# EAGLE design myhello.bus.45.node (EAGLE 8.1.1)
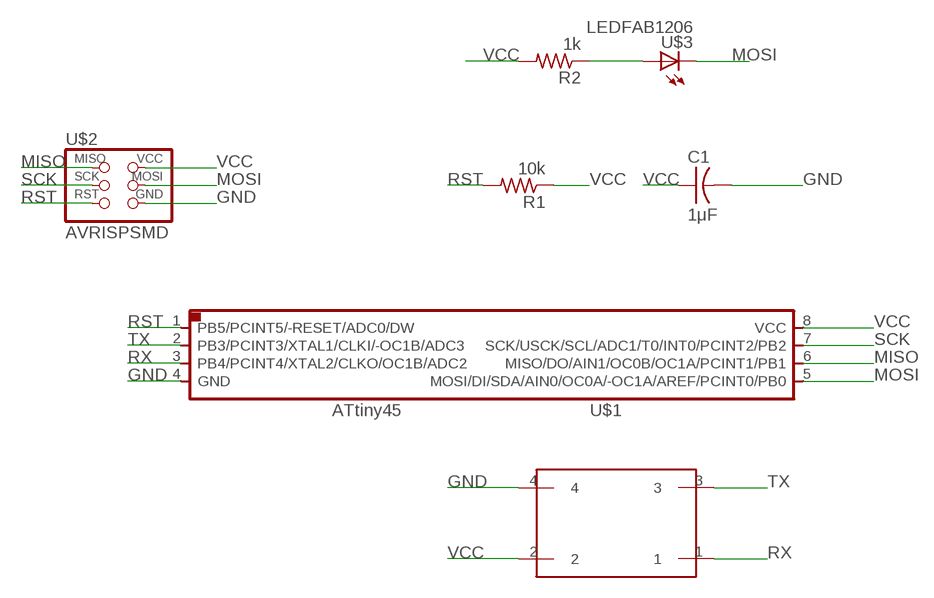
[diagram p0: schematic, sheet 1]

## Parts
C1  1μF  CAP-US1206FAB  [C1206FAB]
R1  10k  RES-US1206FAB  [R1206FAB]
R2  1k  RES-US1206FAB  [R1206FAB]
U$1  ATTINY45SI  [SOIC8]
U$2  AVRISPSMD  [2X03SMD]
U$3  LEDFAB1206  [LED1206FAB]
U$4  4PINHEADER2X2  [2X02SMD]

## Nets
GND: C1.2 U$1.4(GND) U$2.6(GND) U$4.4
MISO: U$1.6(MISO/DO/AIN1/OC0B/OC1A/PCINT1/PB1) U$2.1(MISO)
MOSI: U$1.5(MOSI/DI/SDA/AIN0/OC0A/-OC1A/AREF/PCINT0/PB0) U$2.4(MOSI) U$3.2(C)
N$20: R2.1 U$3.1(A)
RST: R1.2 U$1.1(PB5/PCINT5/-RESET/ADC0/DW) U$2.5(RST)
RX: U$1.3(PB4/PCINT4/XTAL2/CLKO/OC1B/ADC2) U$4.1
SCK: U$1.7(SCK/USCK/SCL/ADC1/T0/INT0/PCINT2/PB2) U$2.3(SCK)
TX: U$1.2(PB3/PCINT3/XTAL1/CLKI/-OC1B/ADC3) U$4.3
VCC: C1.1 R1.1 R2.2 U$1.8(VCC) U$2.2(VCC) U$4.2

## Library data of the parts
C1 = fab:CAP-US
R1 R2 = fab:RES-US: Resistor (US Symbol)
U$1 = fab:ATTINY45
U$2 = fab:AVRISP
U$3 = fab:LED: LED
U$4 = 4pinHeader2X2:4PINHEADER2X2

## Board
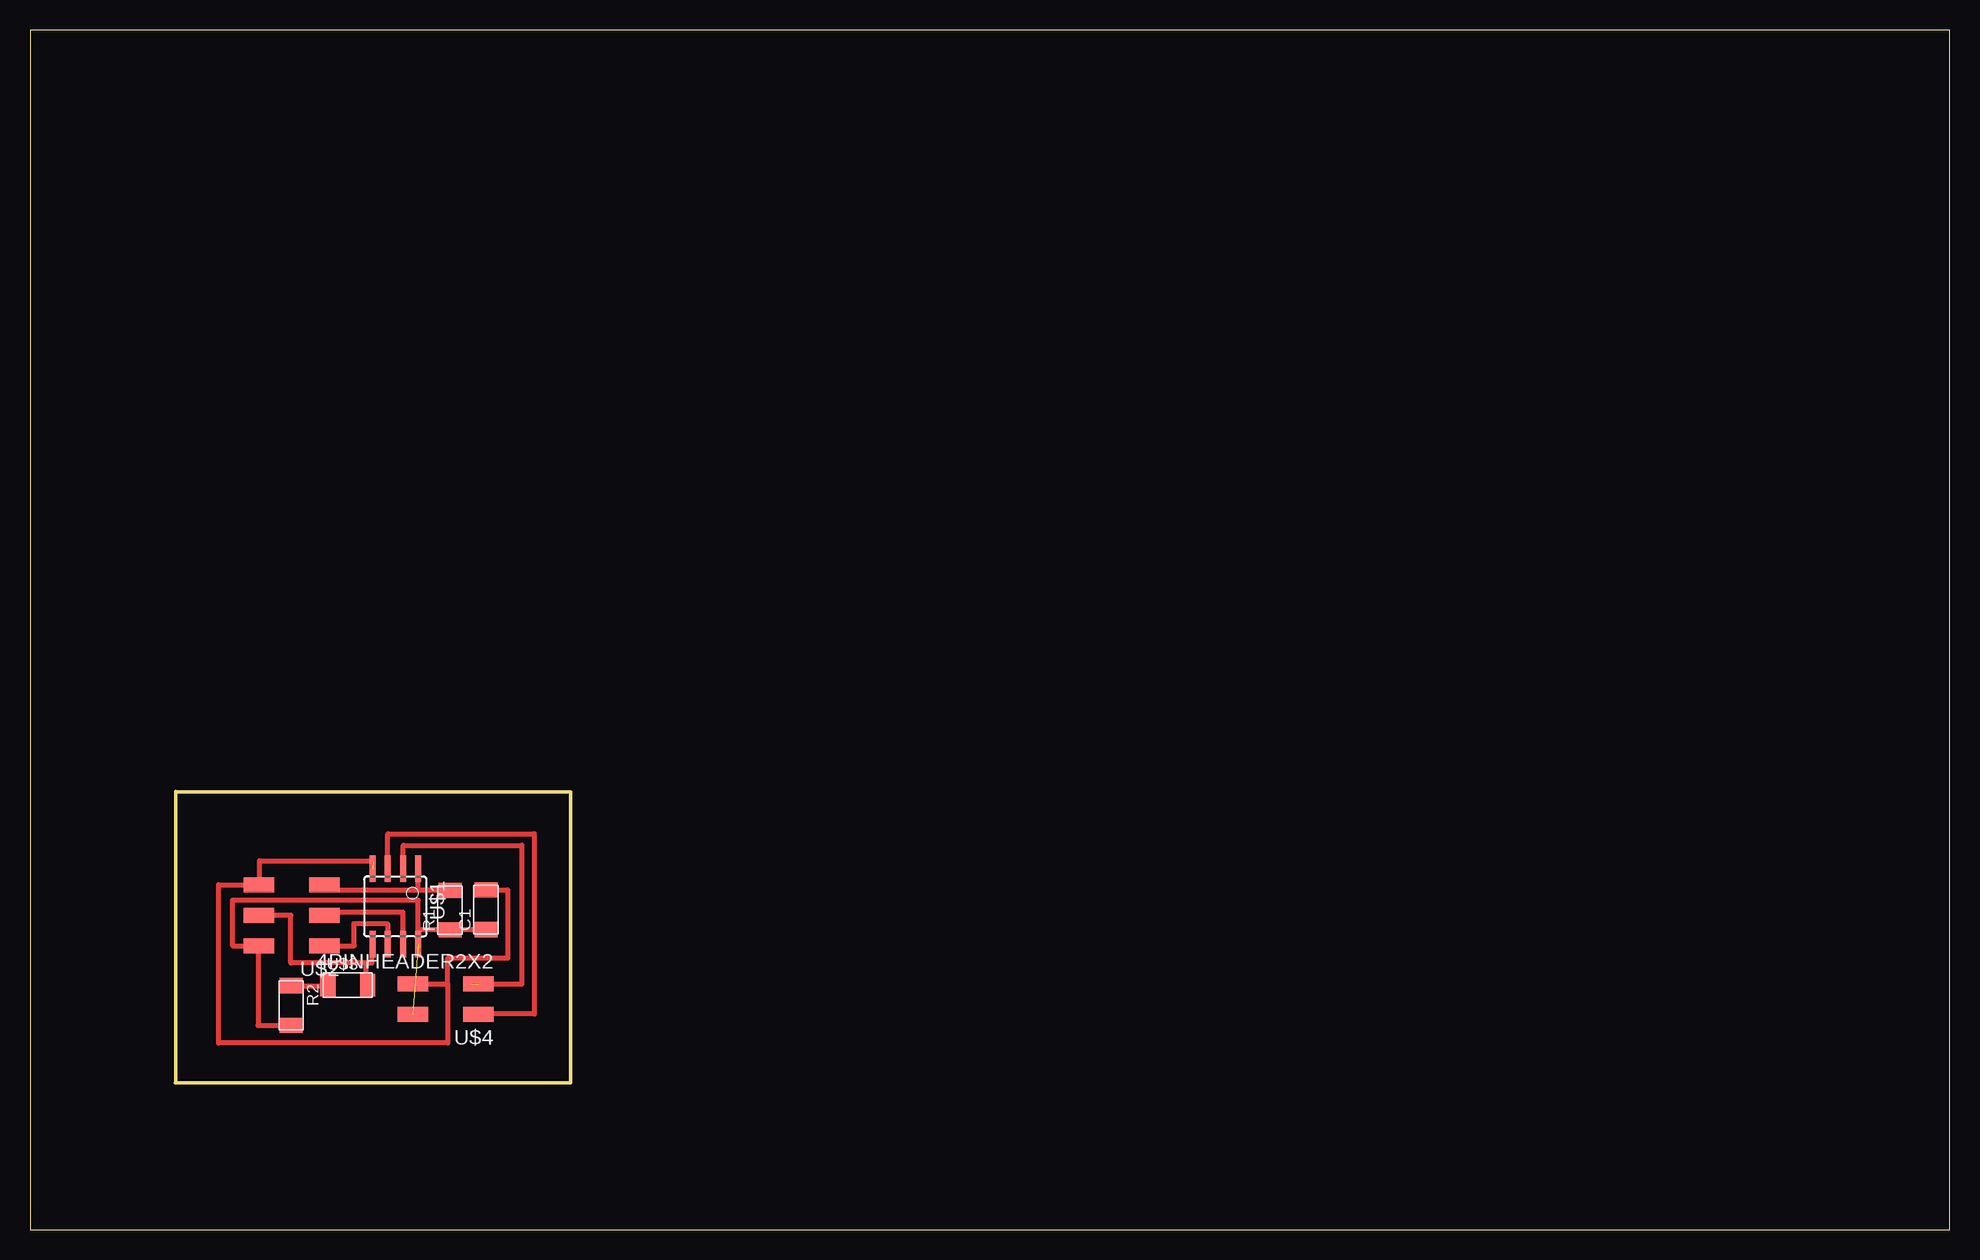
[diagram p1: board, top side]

Size 160 x 100 mm. Coordinates in mm from the lower left corner, seen from the top.
Outline: 12.23,36.49 45.07,36.49 45.07,12.23 12.16,12.23
Outline: 12.12,12.23 12.16,12.23
Outline: 12.16,12.23 12.16,36.53
Outline: 0,0 160,0 160,100 0,100 0,0
Copper layers (1*16): Top 0.035mm / dielectric 1.5mm / Bottom 0.035mm
Design rules "default": minimum track width 10mil, minimum drill 24mil, track to track 8mil, track to pad 8mil, pad to pad 8mil, via to via 8mil, smd to smd 8mil, copper to edge 40mil, drill to drill 8mil, minimum pad ring 10mil, minimum via ring 8mil, stop-mask expansion 4mil, vias tented up to drill 0mil, thermal gap 10mil

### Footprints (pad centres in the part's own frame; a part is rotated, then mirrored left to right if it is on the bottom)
C1206FAB = smd 1.27 x 1.905: 1 -1.651,0; 2 1.651,0
R1206FAB = smd 1.27 x 1.905: 1 -1.651,0; 2 1.651,0
SOIC8 = smd 0.5 x 2.2: 1 -1.905,-3.154; 2 -0.645,-3.154; 3 0.625,-3.154; 4 1.895,-3.154; 5 1.905,3.154; 6 0.635,3.154; 7 -0.635,3.154; 8 -1.905,3.154
2X03SMD = smd 2.54 x 1.27: 1 -2.54,2.54; 2 2.92,2.54; 3 -2.54,0; 4 2.92,0; 5 -2.54,-2.54; 6 2.92,-2.54
LED1206FAB = smd 1.27 x 1.905: 1 -1.651,0; 2 1.651,0
2X02SMD = smd 2.54 x 1.27: 1 -2.54,1.27; 2 2.92,1.27; 3 -2.54,-1.27; 4 2.92,-1.27

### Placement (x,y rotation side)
C1  38.01,26.66 90 top
R1  35.01,26.63 90 top
R2  21.77,18.68 270 top
U$1  30.45,26.93 180 top
U$2  21.99,26.19 180 top
U$3  26.49,20.38 0 top
U$4  34.83,19.2 180 top

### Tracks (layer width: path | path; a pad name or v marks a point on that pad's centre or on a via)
GND  (1 unrouted)
  Top 0.406: C1.2 39.83,28.31 | 39.85,28.31 39.83,28.31 | 39.83,28.31 39.83,22.62 34.82,22.62 34.82,20.39 | 34.82,20.39 34.82,15.56 15.71,15.56 15.71,28.73 U$2.6 19.14,28.73 19.14,30.73 28.61,30.73 28.61,30.67 | U$4.4 34.82,20.47 34.82,20.39
MISO
  Top 0.406: U$2.1 27.04,23.65 27.02,25.52 29.8,25.52 U$1.6
MOSI
  Top 0.406: U$1.5 28.49,23.78 28.49,22.21 28,22.21 | 28,22.21 21.74,22.21 21.74,26.19 U$2.4 | U$3.2 28,20.38 28,22.21
N$20
  Top 0.406: R2.1 24.84,20.33 U$3.1
RST
  Top 0.406: R1.2 32.35,28.28 | 32.35,28.28 24.51,28.28 U$2.5 | 32.35,28.28 U$1.1
RX
  Top 0.406: U$1.3 29.82,32.98 42.03,32.98 42.03,17.96 37.37,17.96 U$4.1
SCK
  Top 0.406: U$1.7 31.09,26.44 24.53,26.44 U$2.3
TX  (1 unrouted)
  Top 0.406: U$1.2 31.12,30.08 31.12,32.03 40.99,32.03 40.99,20.45 36.8,20.45 36.8,20.39
VCC  (1 unrouted)
  Top 0.406: 32.35,24.98 32.35,27.47 16.88,27.47 16.88,23.65 U$2.2 19.02,23.65 19.02,17.01 21.77,17.01 R2.2 | 32.35,24.98 U$1.8 | 32.35,24.98 R1.1 38.01,24.98 C1.1 37.75,25.01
